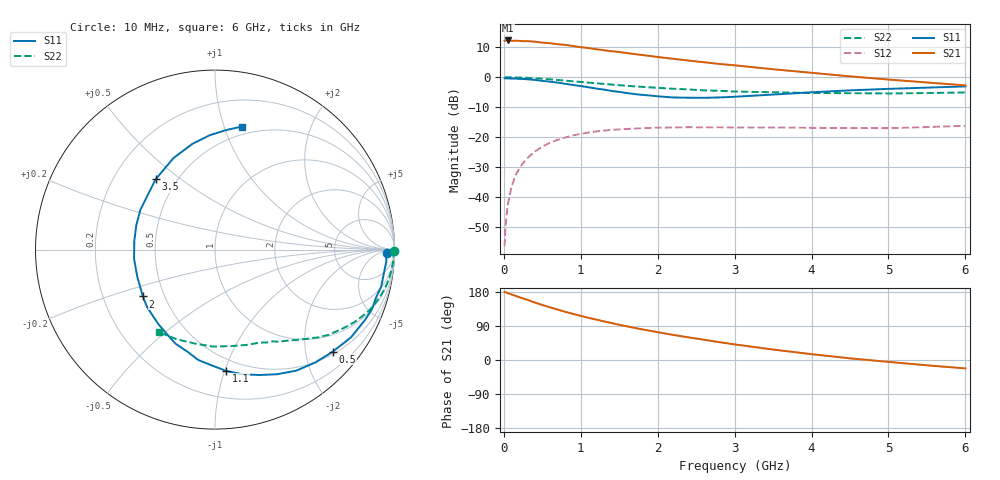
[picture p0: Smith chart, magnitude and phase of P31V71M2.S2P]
! SIEMENS Small Signal Semiconductors
! BFP181
! Si NPN RF Bipolar Junction Transistor in SOT143
! VCE = 1.75 V  IC = 1.2 mA
! Common Emitter S-Parameters:  March  1996
# GHz  S  MA  R  50
!  f  S11  S21  S12  S22
! GHz  MAG  ANG  MAG  ANG  MAG  ANG  MAG  ANG
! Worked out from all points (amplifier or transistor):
!   36 points, 10 MHz to 6 GHz, reference 50 ohm
!   highest |S21| = 12.3 dB at 50 MHz (marker M1)
!   |S21| within 3 dB of that: start of sweep to 1.222 GHz
!   unconditionally stable (mu >= 1): 2.847 GHz to end of sweep
!   at 250 MHz: K = 0.10, MSG = 20.4 dB, |S12| = -28.7 dB
!   at 1.4 GHz: K = 0.54, MSG = 13.2 dB, |S12| = -17.6 dB
!   at 6 GHz: K = 1.26, MAG = 3.7 dB, |S12| = -16.2 dB
!   S11 on the Smith chart (normalised r, x): 10 MHz: 39, -15; 500 MHz: 0.56, -2.58; 1.1 GHz: 0.40, -1.01; 2 GHz: 0.38, -0.26; 3.5 GHz: 0.38, +0.41; 6 GHz: 0.43, +1.15
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0.01  0.9559 -1.0  4.068 179.5  0.0015 85.9  0.998 -0.3
0.02  0.9549 -1.8  4.105 179.3  0.003 90.0  0.9952 -0.7
0.05  0.9567 -4.0  4.112 176.5  0.0073 88.5  0.9957 -2.0
0.1  0.9497 -8.4  4.037 173.0  0.0147 85.3  0.9948 -3.8
0.15  0.949 -12.5  4.083 169.4  0.0226 80.9  0.9913 -5.8
0.2  0.9362 -16.6  4.045 165.8  0.0296 79.5  0.987 -7.7
0.3  0.9234 -25.1  4.007 159.3  0.0437 74.0  0.9764 -11.4
0.4  0.9019 -32.8  3.929 151.8  0.0569 69.2  0.9607 -15.1
0.5  0.8683 -40.9  3.78 145.2  0.069 64.0  0.9426 -18.4
0.6  0.8415 -48.3  3.7 139.0  0.0804 59.2  0.9222 -21.7
0.8  0.7754 -63.6  3.469 127.0  0.0985 51.0  0.8762 -27.4
1.1  0.6789 -84.7  3.072 111.2  0.1188 39.9  0.8106 -34.5
1.5  0.5684 -112.8  2.641 92.9  0.1341 29.1  0.7342 -42.1
1.8  0.5059 -133.5  2.347 80.7  0.1406 23.0  0.6894 -46.6
2  0.4793 -147.0  2.177 73.5  0.1435 19.4  0.6647 -49.4
2.2  0.4587 -160.8  2.031 66.2  0.1443 16.2  0.6412 -52.5
2.8  0.4588 162.9  1.666 47.1  0.1457 9.2  0.5925 -60.9
3.5  0.5126 130.2  1.358 27.6  0.1445 4.5  0.5595 -71.7
4  0.5601 114.4  1.184 15.4  0.1425 2.4  0.5445 -81.1
4.5  0.6026 102.0  1.033 4.4  0.141 0.9  0.5403 -91.4
5.5  0.669 84.6  0.816 -14.0  0.1467 3.0  0.5431 -113.0
6  0.7021 77.6  0.73 -22.2  0.1543 2.8  0.5569 -124.1
